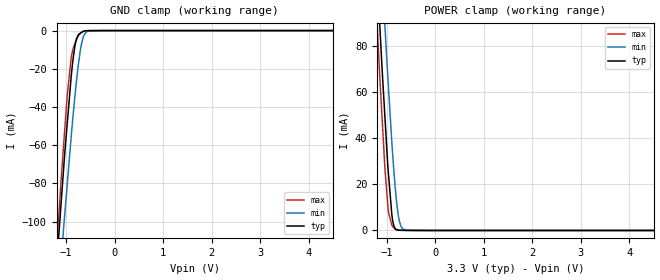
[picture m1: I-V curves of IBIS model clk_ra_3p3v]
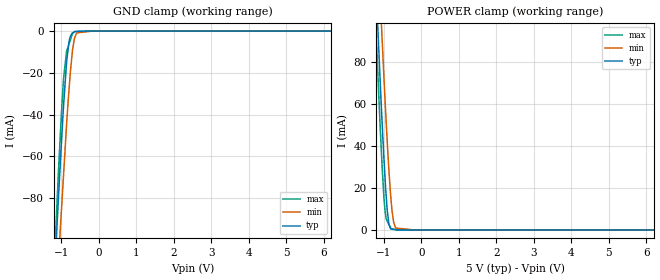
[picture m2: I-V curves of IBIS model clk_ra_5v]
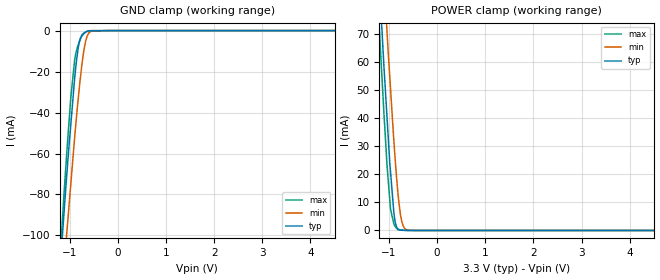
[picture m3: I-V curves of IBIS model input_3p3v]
|Texas Instruments Incorporated
| 10 Bit, 8 MSPS ADC W/Dual Channel, Parallel DSP/uP Interface,
| 16X FIFO, Channel AutoScan, Low Power
| Marketing part#   Digital Voltage Range   Package-type   #pins
| THS10082IDA   3.0V - 5.25V   TSSOP   32
| THS10082IDAG4   3.0V - 5.25V   TSSOP   32
[IBIS Ver]   4.0
[File name]   ths10082.ibs
[File Rev]   1.0
[Date]   12/27/2011
[Source]
| Texas Instruments Incorporated.
| Analog-eLab Design Center, HPA
| 12500 TI Blvd
| Dallas, TX -75243
| e-mail: elab_scm_ibis@list.ti.com
[Notes]   Revision History:
| Rev 1.0: 12/27/2011
| - Initial version of the model
| - Model generated from simulations in TISPICE
| - Model matched to SPICE simulation
| - C_comp although listed in numerical order of value are
|   obtained from varying PVT conditions. For PVT conditions for
|   each specific value refer the buffer description under
|   respective [Model]. IBIS model user is responsible for using
|   appropriate C_comp to simulate for Signal Integrity.
| - Model names with a trailing _3p3 contains the model for
|   3.3V [3.0V and 3.6V]. Model names with a trailing _5 contains
|   the model for 5.0V [4.75V and 5.25V].
[Disclaimer]
| This model is designed as an aid for customers of Texas Instruments.
| TI and its licensors and suppliers make no warranties, either expressed
| or implied, with respect to this  model, including the warranties of
| merchantability or fitness for a particular purpose. The model is
| provided solely on an "as is" basis. The entire risk as to its quality
| and performance is with the customer.
[Copyright]
 (C) Copyright 2012 Texas Instruments Incorporated.All rights reserved.
|   THS10082
[Component]   THS10082
[Manufacturer]   TI
[Package]   |32 TSSOP   -  DA package
|   typ   min   max
R_pkg   0.22349   0.20935   0.24230
L_pkg   3.56109nH   2.82748nH   5.26107nH
C_pkg   0.76313pF   0.65107pF   0.89665pF
[Pin]  signal_name   model_name   R_pin   L_pin   C_pin
1   D0   DB   0.23660   5.10197nH  0.88632pF
2   D1   DB   0.22824   4.15037nH  0.83153pF
3   D2   DB   0.23170   3.54048nH  0.76928pF
4   D3   DB   0.22790   3.45427nH  0.76690pF
5   D4   DB   0.21901   3.21370nH  0.75682pF
6   D5   DB   0.21584   3.07611nH  0.69847pF
7   BVDD   POWER   0.21269   2.91205nH  0.67046pF
8   BGND   GND   0.21047   2.79716nH  0.64638pF
9   D6   DB   0.21377   2.82748nH  0.66907pF
10   D7   DB   0.21458   2.92175nH  0.66849pF
11   D8   DB   0.21614   3.07364nH  0.69753pF
12   D9   DB   0.22067   3.23034nH  0.75697pF
13   RA0   CLK_RA   0.22630   3.43331nH  0.76788pF
14   RA1   CLK_RA   0.23221   3.54819nH  0.76968pF
15   CONV_CLK(_CONVST) CLK_RA   0.22890   4.15953nH  0.83396pF
16   DATA_AV   DATA_AV   0.23697   5.10236nH  0.88787pF
17   DGND   GND   0.23354   5.07864nH  0.88757pF
18   DVDD   POWER   0.22775   4.14883nH  0.83532pF
19   _RD   INPUT   0.22349   3.47204nH  0.77751pF
20   _WR(R/_W)   INPUT   0.21833   3.37323nH  0.76759pF
21   CS1   INPUT   0.21330   3.16831nH  0.75570pF
22   _CS0   INPUT   0.21263   3.05054nH  0.69695pF
23   AVDD   POWER   0.21439   2.92741nH  0.66643pF
24   AGND   GND   0.12364   2.47453nH  0.68936pF
25   REFM   TERM   0.21568   2.83733nH  0.65107pF
26   REFP   TERM   0.21574   2.93112nH  0.67527pF
27   REFOUT   TERM   0.22130   3.11874nH  0.70174pF
28   REFIN   TERM   0.20935   3.13455nH  0.74859pF
29   AINM   TERM   0.21905   3.38287nH  0.72574pF
30   AINP   TERM   0.24112   3.66662nH  0.81322pF
31   _RESET   RESET   0.22953   4.35847nH  0.87055pF
32   OV_FL   OVFL   0.24230   5.26107nH  0.89665pF
1000   thermal_pad   NC   0.00004   0.00163nH  3.26032pF
|   Model Selectors
[Model Selector] CLK_RA
clk_ra_3p3v  3.3V digital input
clk_ra_5v   5.0V digital input
[Model Selector] INPUT
input_3p3v   3.3V digital input
input_5v   5.0V digital input
[Model Selector] RESET
reset_3p3v  3.3V digital input
reset_5v   5.0V digital input
[Model Selector] DB
db_3p3v  3.3V digital 3-state
db_5v   5.0V digital 3-state
[Model Selector] DATA_AV
data_av_3p3v  3.3V digital output
data_av_5v   5.0V digital output
[Model Selector] OVFL
ovfl_3p3v  3.3V digital output
ovfl_5v   5.0V digital output
[Model Selector] TERM
term_3-3V  3.3V nominal termination
term_5-0V  5.0V nominal termination
[Model] term_3-3V
Model_type Terminator
C_comp   1.0e-20F  1.0e-20F  1.0e-20F
|   typ   min   max
[Voltage Range]   3.3V   3.0V   3.6V
[POWER Clamp Reference]   3.3V   3.0V   3.6V
[GND Clamp Reference]   0V   0V   0V
|Ambient Temperature   25   85   -40
|Junction Temperature
[Temperature Range]   27   125   -40
[Model] term_5-0V
Model_type Terminator
C_comp   1.0e-20F  1.0e-20F  1.0e-20F
|   typ   min   max
[Voltage Range]   5.0V   4.75V   5.25V
[POWER Clamp Reference]   5.0V   4.75V   5.25V
[GND Clamp Reference]   0V   0V   0V
|Ambient Temperature   25   85   -40
|Junction Temperature
[Temperature Range]   27   125   -40
| Models and submodels in the file (14): clk_ra_3p3v (Input), clk_ra_5v (Input), input_3p3v (Input), input_5v (Input), reset_3p3v (Input), reset_5v (Input), db_3p3v (I/O), db_5v (I/O), data_av_3p3v (Output), data_av_5v (Output), ovfl_3p3v (Output), ovfl_5v (Output), term_3-3V (Terminator), term_5-0V (Terminator)
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|   clk_3p3v Model
[Model]   clk_ra_3p3v
Model_type   Input
Vinl = 0.6
Vinh = 2
|   typ   min   max
C_comp   1.043e-12   1.039e-12   1.060e-12
[Voltage Range]   3.3   3   3.6
|Ambient Temperature   25   85   -40
|Junction Temperature
[Temperature Range]   27   125   -40
[Power Clamp Reference]   3.3   3   3.6
[GND Clamp Reference]   0   0   0
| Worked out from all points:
|   GND clamp passes 1 mA (typ) near -0.68 V on its own axis
|   POWER clamp passes 1 mA (typ) near -0.83 V on its own axis
[GND Clamp]
|   Voltage   I(typ)   I(min)   I(max)
-3.3V     -998mA     -962.6mA   -1.056A
-1.218V   -129.7mA   -157.8mA   -122.8mA
-1.105V   -90.24mA   -120.4mA   -78.14mA
-1.059V   -74.03mA   -105mA     -61.78mA
-979.2mV  -48.62mA   -80.48mA   -33.71mA
-896.4mV  -23.64mA   -55.02mA   -13.95mA
-821.7mV  -8.157mA   -34.69mA   -6.791mA
-788.7mV  -4.439mA   -26.41mA   -4.605mA
-714mV    -1.471mA   -11.11mA   -1.615mA
-633.6mV  -182.5uA   -2.501mA   -195.1uA
-285mV    -13.98uA   -318nA     -92.94nA
6.6V      0A         0A         0A
[POWER Clamp]
|   Voltage   I(typ)   I(min)   I(max)
-3.3V     1.052A     1.071A     1.051A
-1.28V    144.1mA    185.5mA    123.5mA
-1.152V   91.41mA    132.1mA    69.15mA
-1.037V   48.13mA    87.66mA    25.84mA
-968.4mV  24.84mA    62.73mA    8.065mA
-897.6mV  6.861mA    38.25mA    2.297mA
-858mV    2.215mA    26.46mA    1.161mA
-810mV    493.1uA    14.53mA    237.7uA
-765mV    191.8uA    6.647mA    184.2uA
-714mV    66.85uA    2.058mA    123.5uA
-591mV    55.28uA    69.39uA    15.7uA
6.6V      0A         0A         0A
|   clk_5v Model
[Model]   clk_ra_5v
Model_type   Input
Vinl = 0.6
Vinh = 2.6
|   typ   min   max
C_comp   9.560e-13   9.523e-13   9.597e-13
[Voltage Range]   5   4.75   5.25
|Ambient Temperature   25   85   -40
|Junction Temperature
[Temperature Range]   27   125   -40
[Power Clamp Reference]   5   4.75   5.25
[GND Clamp Reference]   0   0   0
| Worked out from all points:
|   GND clamp passes 1 mA (typ) near -0.71 V on its own axis
|   POWER clamp passes 1 mA (typ) near -0.83 V on its own axis
[GND Clamp]
|   Voltage   I(typ)   I(min)   I(max)
-5V       -1.749A    -1.672A    -1.846A
-1.306V   -162.7mA   -188.3mA   -158.6mA
-1.088V   -83.48mA   -114.4mA   -71.7mA
-1.031V   -64.75mA   -95.98mA   -51.17mA
-939.7mV  -35.76mA   -68.75mA   -22.6mA
-855mV    -13.98mA   -43.38mA   -9.469mA
-760mV    -2.585mA   -19.88mA   -4.35mA
-698.3mV  -901.6uA   -8.695mA   -1.022mA
-640mV    -213.3uA   -3.025mA   -237.7uA
-593.8mV  -169.5uA   -914.2uA   -220.5uA
-190mV    0A         -23.35nA   -70.56uA
10V       0A         0A         0A
[POWER Clamp]
|   Voltage   I(typ)   I(min)   I(max)
-5V       1.848A     1.855A     1.856A
-1.306V   156mA      195.4mA    136.1mA
-1.113V   77.27mA    117.3mA    55.22mA
-1.054V   54.34mA    94.27mA    33.4mA
-966mV    24.2mA     61.42mA    8.882mA
-910mV    9.471mA    42.48mA    4.279mA
-860mV    2.461mA    27.4mA     2.449mA
-803.3mV  600.5uA    13.57mA    372.2uA
-736.2mV  360.3uA    3.552mA    231.3uA
-684mV    172.9uA    934.6uA    121.4uA
-190mV    0A         0A         8.884uA
10V       0A         0A         0A
|   rd_3p3v Model
[Model]   input_3p3v
Model_type   Input
Vinl = 0.6
Vinh = 2
|   typ   min   max
C_comp   1.043e-12   1.039e-12   1.060e-12
[Voltage Range]   3.3   3   3.6
|Ambient Temperature   25   85   -40
|Junction Temperature
[Temperature Range]   27   125   -40
[Power Clamp Reference]   3.3   3   3.6
[GND Clamp Reference]   0   0   0
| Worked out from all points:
|   GND clamp passes 1 mA (typ) near -0.68 V on its own axis
|   POWER clamp passes 1 mA (typ) near -0.83 V on its own axis
[GND Clamp]
|   Voltage   I(typ)   I(min)   I(max)
-3.3V     -935.6mA   -897.7mA   -995.1mA
-1.224V   -123.9mA   -149mA     -118.7mA
-1.112V   -86.46mA   -114.3mA   -77.2mA
-1.062V   -70.38mA   -98.66mA   -59.48mA
-979.2mV  -46.05mA   -75.05mA   -32.84mA
-896.4mV  -22.69mA   -51.46mA   -13.92mA
-821.7mV  -8.032mA   -32.63mA   -6.791mA
-785.4mV  -4.151mA   -24.23mA   -4.431mA
-711mV    -1.434mA   -10.23mA   -1.518mA
-630.3mV  -168.3uA   -2.292mA   -315.6uA
-285mV    -75.61uA   -318nA     -92.94nA
6.6V      0A         0A         0A
[POWER Clamp]
|   Voltage   I(typ)   I(min)   I(max)
-3.3V     822mA      833.2mA    825.8mA
-1.31V    123.6mA    154.4mA    109mA
-1.164V   77.17mA    108.1mA    60.31mA
-1.112V   60.68mA    92.42mA    44.02mA
-1.04V    40.27mA    70.76mA    23.25mA
-968.4mV  20.97mA    50.69mA    7.672mA
-897.6mV  6.234mA    31.56mA    2.289mA
-858mV    2.124mA    22.28mA    1.141mA
-810mV    488.6uA    12.7mA     237.7uA
-735mV    72.91uA    3.267mA    147.3uA
-591mV    9.718uA    69.3uA     15.7uA
6.6V      0A         0A         0A
